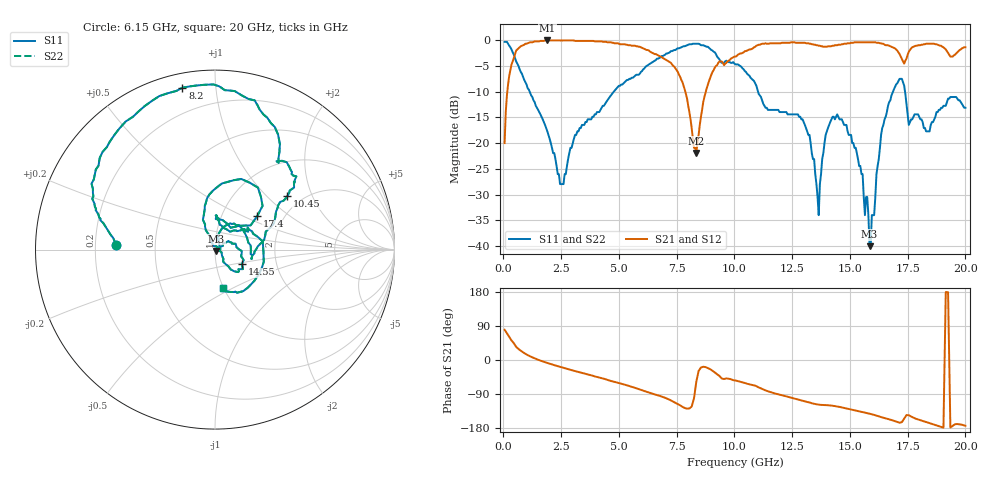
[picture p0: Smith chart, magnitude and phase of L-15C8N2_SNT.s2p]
# MHZ S MA R 50
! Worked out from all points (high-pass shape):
!   400 points, 50 MHz to 20 GHz, reference 50 ohm
!   highest |S21| = -0.09 dB at 1.9 GHz (marker M1); lowest = -21.9 dB at 8.35 GHz (marker M2)
!   |S21| within 3 dB of the highest: 476.3 MHz to 6.746 GHz (6.269 GHz wide, 174 % of centre); 10.1 GHz to 17.19 GHz (7.084 GHz wide, 51.9 % of centre)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
!   lowest |S11| = -40.0 dB at 15.85 GHz (marker M3), VSWR 1.02, Z = 50.6 - j0.769 ohm
!   |S11| at or under -10 dB: 1.134 GHz to 4.781 GHz (3.647 GHz wide, 123 % of centre); 11.02 GHz to 16.87 GHz (5.844 GHz wide, 41.9 % of centre); 17.39 GHz to end of sweep
!   |S22| runs from -40.0 to -0.4 dB; largest |S21 - S12| = 0
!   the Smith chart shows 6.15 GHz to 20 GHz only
!   S11 on the Smith chart (normalised r, x): 6.15 GHz: 0.29, +0.02; 8.2 GHz: 0.07, +0.82; 10.45 GHz: 1.68, +1.33; 14.55 GHz: 1.33, -0.22; 17.4 GHz: 1.47, +0.60; 20 GHz: 0.99, -0.45
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50  0.96 173.8  0.1 79.8  0.1 79.8  0.96 173.8
1900  0.13 91.0  0.99 -7.8  0.99 -7.8  0.13 91.0
3400  0.15 -134.9  0.98 -34.1  0.98 -34.1  0.15 -134.9
6050  0.52 -179.7  0.83 -81.0  0.83 -81.0  0.52 -179.7
6100  0.53 -1.1  0.82 -81.9  0.82 -81.9  0.53 -1.1
6150  0.55 177.4  0.81 -82.8  0.81 -82.8  0.55 177.4
6700  0.66 165.0  0.71 -93.5  0.71 -93.5  0.66 165.0
8200  0.92 101.4  0.11 -112.0  0.11 -112.0  0.92 101.4
8350  0.92 94.1  0.08 -57.3  0.08 -57.3  0.92 94.1
10050  0.58 40.1  0.69 -54.1  0.69 -54.1  0.58 40.1
10450  0.5 36.4  0.78 -60.4  0.78 -60.4  0.5 36.4
13350  0.08 78.2  0.91 -114.2  0.91 -114.2  0.08 78.2
14550  0.17 -28.6  0.9 -123.8  0.9 -123.8  0.17 -28.6
15850  0.01 -49.4  0.95 -141.6  0.95 -141.6  0.01 -49.4
16700  0.25 103.1  0.88 -156.6  0.88 -156.6  0.25 103.1
17400  0.3 38.4  0.63 -150.1  0.63 -150.1  0.3 38.4
19050  0.23 26.5  0.85 -178.6  0.85 -178.6  0.23 26.5
19100  0.23 24.6  0.83 0.3  0.83 0.3  0.23 24.6
19150  0.23 22.7  0.81 179.3  0.81 179.3  0.23 22.7
19300  0.27 -2.3  0.72 0.3  0.72 0.3  0.27 -2.3
19350  0.28 -14.1  0.69 -178.1  0.69 -178.1  0.28 -14.1
20000  0.22 -78.4  0.85 -173.4  0.85 -173.4  0.22 -78.4
